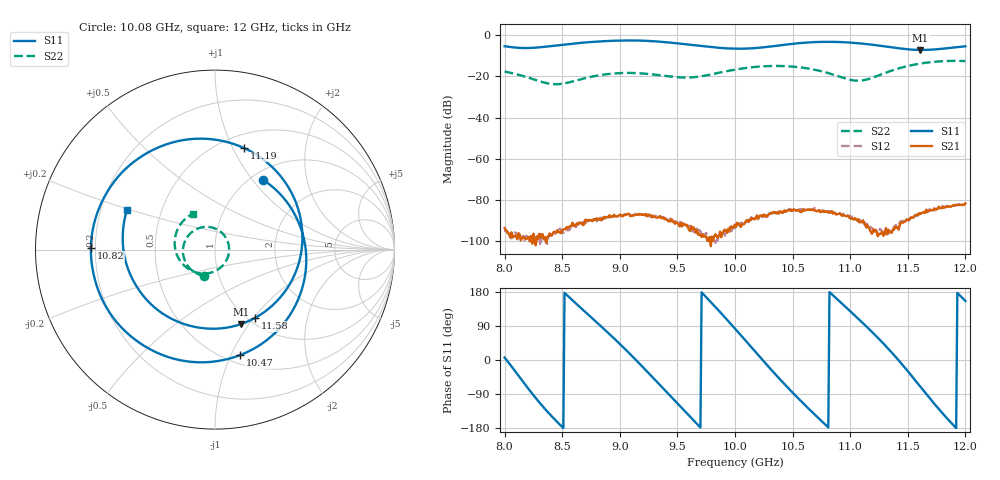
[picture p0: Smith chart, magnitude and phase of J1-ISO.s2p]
!Keysight Technologies,N5234A,MY52241180,A.10.60.03
!Date: Tuesday, May 30, 2023 15:16:39
!Correction: S11(Full 2 Port(1,2))
!S21(Full 2 Port(1,2))
!S12(Full 2 Port(1,2))
!S22(Full 2 Port(1,2))
!S2P File: Measurements: S11, S21, S12, S22:
# Hz S  dB  R 50
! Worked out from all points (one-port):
!   401 points, 8 GHz to 12 GHz, reference 50 ohm
!   lowest |S11| = -7.1 dB at 11.61 GHz (marker M1), VSWR 2.57, Z = 44.7 - j45.9 ohm
!   |S11| at or under -10 dB: nowhere
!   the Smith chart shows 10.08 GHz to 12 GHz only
!   S11 on the Smith chart (normalised r, x): 10.08 GHz: 1.14, +1.13; 10.47 GHz: 0.59, -1.08; 10.82 GHz: 0.18, +0.01; 11.19 GHz: 0.64, +1.11; 11.58 GHz: 1.08, -1.02; 12 GHz: 0.31, +0.19
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8e9  -5.37 6.4  -93.63 154.4  -95.45 147.7  -17.70 116.5
8.29e9  -5.95 -107.7  -98.83 151.0  -97.63 152.2  -22.12 42.3
8.49e9  -4.70 -173.7  -96.13 133.4  -94.74 132.9  -23.63 -36.7
8.67e9  -3.67 135.0  -91.20 91.3  -91.26 92.0  -21.26 -98.7
8.88e9  -2.85 76.9  -88.56 45.6  -88.88 42.6  -18.95 -150.9
9.08e9  -2.55 18.5  -86.70 -3.7  -87.21 -7.6  -18.30 165.2
9.34e9  -3.11 -63.3  -88.10 -76.1  -87.94 -79.3  -19.37 103.0
9.48e9  -3.83 -108.2  -91.49 -111.9  -90.53 -118.4  -20.28 62.3
9.66e9  -4.97 -165.5  -95.84 -132.4  -94.47 -146.5  -20.28 2.0
1e10  -6.52 82.9  -91.92 -130.5  -93.75 -127.6  -16.71 -94.3
1.008e10  -6.52 55.2  -91.70 -136.5  -90.68 -135.1  -16.01 -112.3
1.028e10  -5.68 -14.1  -88.12 171.1  -86.71 170.8  -14.99 -153.7
1.047e10  -4.38 -76.6  -84.66 126.5  -84.48 121.9  -15.12 168.6
1.067e10  -3.40 -137.5  -84.86 70.3  -84.63 72.7  -16.51 127.0
1.082e10  -3.20 179.3  -86.17 29.6  -85.69 29.7  -18.56 90.5
1.102e10  -3.67 123.1  -88.92 -11.9  -88.10 -13.0  -21.86 20.6
1.119e10  -4.61 73.8  -96.34 -43.4  -93.67 -35.9  -20.68 -53.9
1.134e10  -5.74 26.6  -95.64 -18.9  -94.74 -17.2  -17.56 -102.1
1.158e10  -7.11 -59.5  -87.09 -36.6  -87.68 -38.5  -14.03 -157.3
1.161e10  -7.14 -70.8  -86.75 -41.1  -86.34 -42.3  -13.75 -163.3
1.183e10  -6.41 -150.4  -83.44 -95.8  -82.98 -94.9  -12.54 154.1
1.2e10  -5.38 155.8  -81.75 -141.2  -81.84 -139.5  -12.56 122.0
